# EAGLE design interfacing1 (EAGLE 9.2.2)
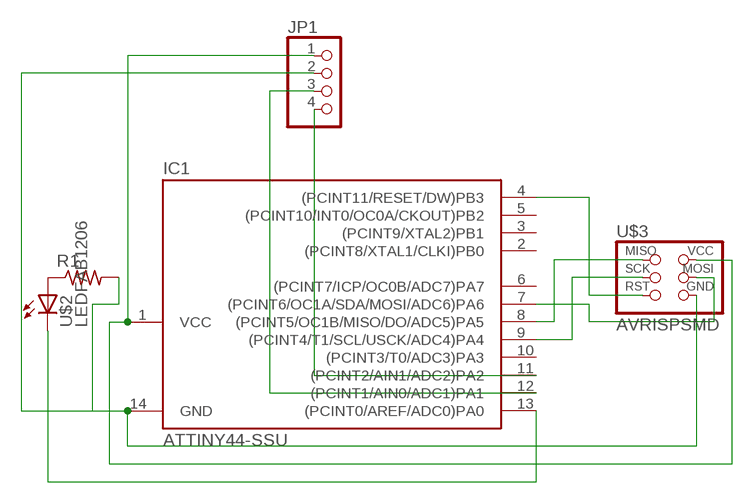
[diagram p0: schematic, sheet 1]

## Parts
IC1  ATTINY44-SSU  [SOIC14]
JP1  PINHD-1X4  [1X04]
R1  RES-US1206FAB  [R1206FAB]
U$2  LEDFAB1206  [LED1206FAB]
U$3  AVRISPSMD  [2X03SMD]

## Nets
N$1: IC1.4((PCINT11/RESET/DW)PB3) U$3.5(RST)
N$2: R1.1 U$2.1(A)
N$3: IC1.9((PCINT4/T1/SCL/USCK/ADC4)PA4) U$3.3(SCK)
N$4: IC1.8((PCINT5/OC1B/MISO/DO/ADC5)PA5) U$3.1(MISO)
N$5: IC1.7((PCINT6/OC1A/SDA/MOSI/ADC6)PA6) U$3.4(MOSI)
N$6: IC1.14(GND) JP1.2 R1.2 U$3.6(GND)
N$7: IC1.1(VCC) JP1.1 U$3.2(VCC)
N$8: IC1.13((PCINT0/AREF/ADC0)PA0) U$2.2(C)
N$9: IC1.12((PCINT1/AIN0/ADC1)PA1) JP1.3
N$10: IC1.11((PCINT2/AIN1/ADC2)PA2) JP1.4
Unconnected: IC1.2((PCINT8/XTAL1/CLKI)PB0) IC1.3((PCINT9/XTAL2)PB1) IC1.5((PCINT10/INT0/OC0A/CKOUT)PB2) IC1.6((PCINT7/ICP/OC0B/ADC7)PA7) IC1.10((PCINT3/T0/ADC3)PA3)

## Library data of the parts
IC1 = fab:ATTINY44
JP1 = pinhead:PINHD-1X4: PIN HEADER
R1 = fab:RES-US: Resistor (US Symbol)
U$2 = fab:LED: LED
U$3 = fab:AVRISP

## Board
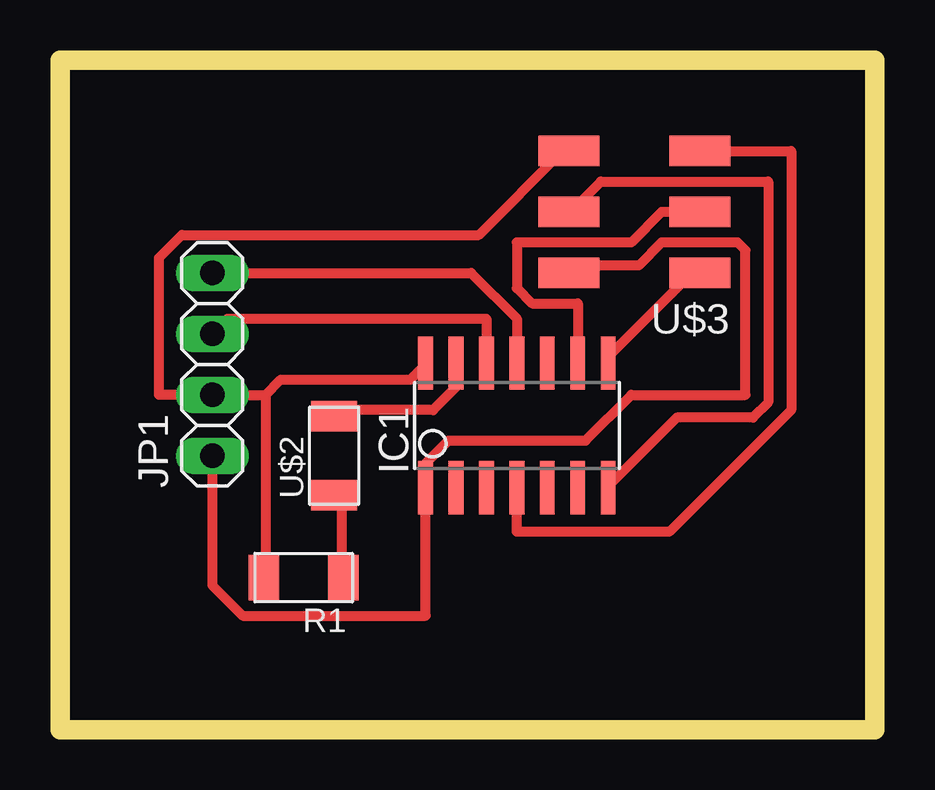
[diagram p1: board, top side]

Size 33.96 x 27.93 mm. Coordinates in mm from the lower left corner, seen from the top.
Outline: 0,0 33.96,0 33.96,27.93 0,27.93 0,0
Copper layers (1*16): Top 0.035mm / dielectric 1.5mm / Bottom 0.035mm
Design rules "default *": minimum track width 16mil, minimum drill 0.35mm, track to track 16mil, track to pad 16mil, pad to pad 16mil, via to via 16mil, smd to smd 16mil, copper to edge 40mil, drill to drill 6mil, minimum pad ring 10mil, minimum via ring 8mil, stop-mask expansion 4mil, vias tented up to drill 0mil, thermal gap 10mil

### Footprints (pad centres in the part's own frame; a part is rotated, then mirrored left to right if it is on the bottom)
SOIC14 = smd 0.61 x 2.21: 1 -3.81,-2.603; 2 -2.54,-2.603; 3 -1.27,-2.603; 4 0,-2.603; 5 1.27,-2.603; 6 2.54,-2.603; 7 3.81,-2.603; 8 3.81,2.603; 9 2.54,2.603; 10 1.27,2.603; 11 0,2.603; 12 -1.27,2.603; 13 -2.54,2.603; 14 -3.81,2.603
1X04 = drill 1.016 long: 1 -3.81,0; 2 -1.27,0; 3 1.27,0; 4 3.81,0
R1206FAB = smd 1.27 x 1.905: 1 -1.651,0; 2 1.651,0
LED1206FAB = smd 1.27 x 1.905: 1 -1.651,0; 2 1.651,0
2X03SMD = smd 2.54 x 1.27: 1 -2.54,2.54; 2 2.92,2.54; 3 -2.54,0; 4 2.92,0; 5 -2.54,-2.54; 6 2.92,-2.54

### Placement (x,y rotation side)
IC1  19.05,12.7 0 top
JP1  6.35,15.24 90 top
R1  10.16,6.35 180 top
U$2  11.43,11.43 90 top
U$3  24.13,21.59 180 top

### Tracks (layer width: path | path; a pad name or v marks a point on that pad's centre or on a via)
N$1
  Top 0.406: IC1.4 19.05,8.26 25.4,8.26 30.48,13.34 30.48,24.13 U$3.5
N$2
  Top 0.406: R1.1 11.75,6.35 11.75,9.52 11.43,9.52 U$2.1
N$3
  Top 0.406: IC1.9 21.59,17.78 19.68,17.78 19.05,18.41 19.05,20.32 23.81,20.32 25.08,21.59 U$3.3
N$4
  Top 0.406: U$3.1 26.35,19.05 22.86,15.56 IC1.8
N$5
  Top 0.406: IC1.7 22.86,10.16 25.72,13.02 28.89,13.02 29.53,13.65 29.53,22.86 22.54,22.86 21.27,21.59 U$3.4
N$6
  Top 0.406: 8.57,13.97 8.57,6.35 R1.2 | 8.57,13.97 JP1.2 4.13,13.97 4.13,19.69 5.08,20.64 17.46,20.64 20.95,24.13 U$3.6 | 8.57,13.97 9.21,14.6 14.6,14.6 15.24,15.24 IC1.14
N$7
  Top 0.406: JP1.1 6.35,6.03 7.62,4.76 15.24,4.76 IC1.1 15.24,11.11 16.19,12.06 21.91,12.06 23.81,13.97 28.57,13.97 28.57,20 28.26,20.32 25.08,20.32 24.13,19.37 21.59,19.37 21.27,19.05 U$3.2
N$8
  Top 0.406: IC1.13 16.51,14.29 15.56,13.34 11.43,13.34 U$2.2
N$9
  Top 0.406: IC1.12 17.78,17.15 6.98,17.15 JP1.3
N$10
  Top 0.406: IC1.11 19.05,17.15 17.14,19.05 JP1.4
